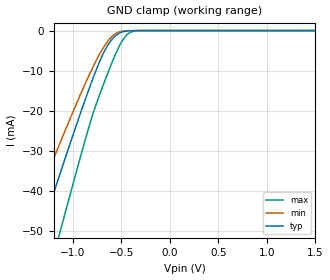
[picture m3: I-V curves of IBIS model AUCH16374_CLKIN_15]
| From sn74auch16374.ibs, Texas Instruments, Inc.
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[Model]   AUCH16374_CLKIN_15
Model_type  Input
Vinl=0.49
Vinh=1.04
| variable   typ   min   max
C_comp   2.47pF   2.05pF   2.79pF
[Temperature Range]   40   100   -40
| Ambient temperature   25   85   -40
[Voltage range]   1.5   1.4   1.6
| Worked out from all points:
|   GND clamp passes 1 mA (typ) near -0.55 V on its own axis
[GND Clamp]
| AUCH16374_CLKIN_15
|   Voltage   I(typ)   I(min)   I(max)
-3.6V     -222.3mA   -186.1mA   -267.5mA
-1.505V   -63.42mA   -50.72mA   -83.44mA
-1.325V   -49.94mA   -39.61mA   -67.39mA
-1.17V    -38.46mA   -30.25mA   -53.55mA
-1.12V    -34.79mA   -27.28mA   -49.08mA
-840mV    -14.98mA   -11.48mA   -24.46mA
-695mV    -6.114mA   -4.621mA   -14.06mA
-570mV    -1.487mA   -911.6uA   -6.381mA
-495mV    -364.6uA   -178.8uA   -2.692mA
-430mV    -73.19uA   -34.73uA   -776.9uA
-280mV    -781.4nA   -556.3nA   -5.358uA
1.5V      165.9pA    258.5pA    172.1pA
